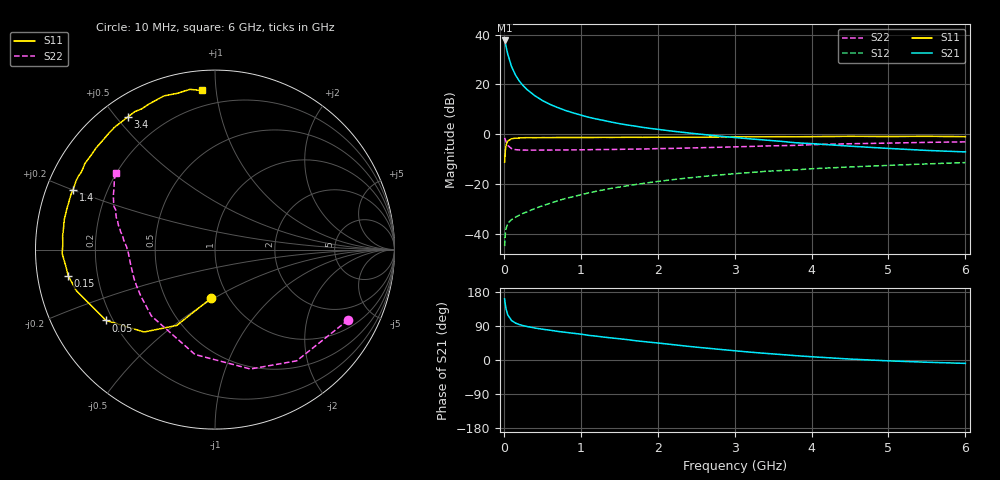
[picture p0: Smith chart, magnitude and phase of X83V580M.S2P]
! SIEMENS Small Signal Semiconductors
! BFP136W
! Si NPN RF Bipolar Junction Transistor in SOT343
! VCE = 3.5 V  IC = 80 mA
! Common Emitter S-Parameters:  September  1994
# GHz  S  MA  R  50
!  f  S11  S21  S12  S22
! GHz  MAG  ANG  MAG  ANG  MAG  ANG  MAG  ANG
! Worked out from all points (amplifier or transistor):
!   40 points, 10 MHz to 6 GHz, reference 50 ohm
!   highest |S21| = 37.6 dB at 10 MHz (marker M1)
!   |S21| within 3 dB of that: start of sweep to 32.89 MHz
!   unconditionally stable (mu >= 1): 571.9 MHz to 2.888 GHz
!   at 200 MHz: K = 0.65, MSG = 27.0 dB, |S12| = -32.6 dB
!   at 1.5 GHz: K = 1.10, MAG = 10.8 dB, |S12| = -21.3 dB
!   at 6 GHz: K = 0.96, MSG = 2.1 dB, |S12| = -11.4 dB
!   S11 on the Smith chart (normalised r, x): 10 MHz: 0.83, -0.49; 50 MHz: 0.17, -0.29; 150 MHz: 0.09, -0.09; 1.4 GHz: 0.08, +0.20; 3.4 GHz: 0.08, +0.54; 6 GHz: 0.11, +0.92
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0.01  0.2733 -94.9  76.29 161.3  0.0056 68.7  0.8386 -27.9
0.02  0.4735 -116.8  66.27 145.3  0.01 59.4  0.7689 -53.7
0.03  0.6057 -130.7  56.6 133.7  0.0128 50.3  0.6938 -73.5
0.05  0.7244 -147.0  40.9 119.4  0.016 39.6  0.595 -100.8
0.1  0.8061 -163.5  22.81 104.3  0.0191 36.1  0.512 -133.8
0.15  0.831 -170.0  15.56 97.6  0.0213 38.1  0.4879 -147.9
0.2  0.8363 -173.7  11.71 93.6  0.0235 39.7  0.4811 -155.7
0.25  0.845 -176.6  9.457 90.7  0.0256 42.2  0.4789 -160.6
0.3  0.8516 -178.5  7.906 88.5  0.0273 44.6  0.4768 -164.0
0.4  0.8484 177.7  5.956 84.5  0.0319 48.7  0.4766 -168.4
0.5  0.8524 174.9  4.749 81.3  0.0362 51.8  0.4778 -171.4
0.6  0.8518 172.9  3.963 78.6  0.0407 54.2  0.4785 -173.3
0.7  0.8541 170.2  3.417 75.5  0.0457 56.5  0.4801 -174.8
0.9  0.8553 166.6  2.675 70.6  0.0552 58.1  0.4822 -177.3
1.1  0.856 162.2  2.187 65.1  0.0657 59.1  0.4864 -179.0
1.4  0.858 157.1  1.745 58.2  0.0815 59.0  0.4913 178.6
2.2  0.8677 143.2  1.143 40.5  0.1218 54.6  0.5164 172.6
3.2  0.8817 126.3  0.803 20.8  0.1689 45.7  0.5647 163.8
3.4  0.8845 123.3  0.76 17.5  0.1787 43.7  0.5783 162.0
4.5  0.9024 108.4  0.573 2.5  0.2189 33.6  0.6405 152.2
5.5  0.9037 98.9  0.47 -5.9  0.252 25.8  0.6829 145.2
6  0.8895 94.7  0.439 -8.9  0.2683 21.5  0.699 142.2
